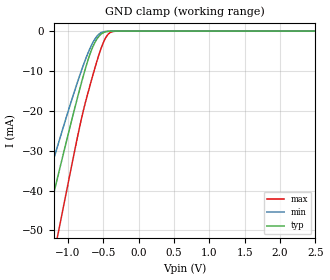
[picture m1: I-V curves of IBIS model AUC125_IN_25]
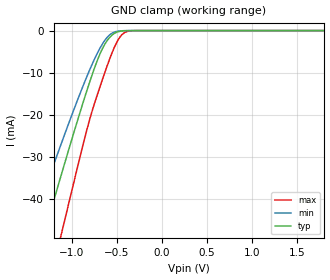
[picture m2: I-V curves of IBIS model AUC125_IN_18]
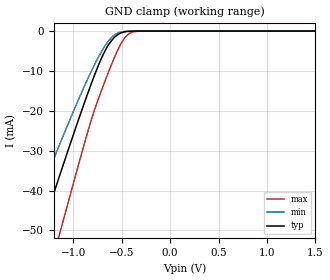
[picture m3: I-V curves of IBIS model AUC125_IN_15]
| TEXAS INSTRUMENTS INCORPORATED
| Standard Linear and Logic Group
| IBIS Model of SN74AUC125
| Quadruple Bus Buffer Gate with 3-state Outputs
| This file contains package information for the following:
|  QFN 14-pin (RGY) package as [Component] AUC125_RGY
| This device can be powered at the following Vccs:
|  2.5 volt Vcc
|  1.8 volt Vcc
|  1.5 volt Vcc
|  1.2 volt Vcc
|  0.8 volt Vcc
| This file provides unique models under the [Model Selector] for each Vcc.
| For operation at a specific Vcc, select the appropriate model after each
| [Model Selector] keyword.
[IBIS Ver]   3.2
[Comment char]  |_char
[File Name]   sn74auc125.ibs
[File Rev]   1.1 | x_die
[Date]   September 12, 2003
[Source]   Data created from TI-SPICE simulations at TI-SLL.
[Notes]   The following is an IBIS list for the AUC125.
   Please contact sllibis@ti.com with questions and
   comments concerning SLL IBIS models.
   - Power clamp data deleted as there is no power-clamp diode.
   - End point warning due to AC and DC mismatch.
   - Non-monotonic data in pullup and pulldown due to
   feedback circuit.
[Disclaimer] Property of Texas Instruments Incorporated.  Unauthorized
   reproduction and/or distribution is strictly prohibited.
   This product is protected under copyright law.
   Created  2003, (C) Copyright  2003, Texas Instruments
   Incorporated, All Rights Reserved
   UNLESS THERE IS A SIGNED, WRITTEN AGREEMENT TO THE
   CONTRARY, TEXAS INSTRUMENTS (TI) IS PROVIDING THE IBIS
   MODELS  AND WITHOUT ANY WARRANTY, EXPRESSED OR
   IMPLIED.  TI assumes no liability for:
   1) the accuracy of the IBIS models provided to your
   company;
   2) the proper functioning of these IBIS Models in your
   design or for any resulting applications; or
   3) infringement of patents, copyrights or intellectual
   property rights resulting from your use of these IBIS
   models.
   TI provides IBIS Models as a service to our customers.
   You and your company shall not distribute, sell or give
   these models to anyone else without prior written
   permission from TI.
   TI reserves the right to make changes to our products or
   to discontinue any semiconductor product or service
   without notice, and advises our customers to obtain the
   latest version of relevant information to verify, before
   placing orders, that the information being relied on is
   current.
   Please be aware that your receipt and use of the IBIS
   information provided shall serve as acceptance of these
   terms and conditions.  If you do not accept these terms,
   you should return or destroy the IBIS models and any
   other accompanying information immediately.
| Component AUC125_RGY 14-pin QFN
[Component]   AUC125_RGY
[Manufacturer]   Texas Instruments, Inc.
[Package]
|   typ   min   max
R_pkg   2.900e-02   2.300e-02   4.100e-02
L_pkg   7.730e-10   6.570e-10   9.980e-10
C_pkg   1.360e-13   1.150e-13   1.560e-13
[Pin]   signal_name   model_name   R_pin   L_pin   C_pin
1   1NOE   AUC125_IN_OE   2.700e-02   8.310e-10   1.300e-13
2   1A   AUC125_IN   2.700e-02   8.660e-10   1.350e-13
3   1Y   AUC125_OUT   4.100e-02   9.980e-10   1.560e-13
4   2NOE   AUC125_IN_OE   3.100e-02   7.670e-10   1.420e-13
5   2A   AUC125_IN   3.100e-02   7.650e-10   1.420e-13
6   2Y   AUC125_OUT   3.100e-02   7.830e-10   1.440e-13
7   GND   GND   3.100e-02   7.810e-10   1.370e-13
8   3Y   AUC125_OUT   2.300e-02   6.570e-10   1.150e-13
9   3A   AUC125_IN   2.300e-02   8.140e-10   1.290e-13
10   3NOE   AUC125_IN_OE   2.800e-02   7.040e-10   1.290e-13
11   4Y   AUC125_OUT   2.700e-02   6.720e-10   1.360e-13
12   4A   AUC125_IN   2.700e-02   6.960e-10   1.380e-13
13   4NOE   AUC125_IN_OE   2.700e-02   7.250e-10   1.400e-13
14   VCC   POWER   3.000e-02   7.630e-10   1.360e-13
| Model AUC125_IN
[Model Selector]   AUC125_IN
AUC125_IN_25   2.5 volt Vcc
AUC125_IN_18   1.8 volt Vcc
AUC125_IN_15   1.5 volt Vcc
AUC125_IN_12   1.2 volt Vcc
AUC125_IN_08   0.8 volt Vcc
| Model AUC125_IN_OE
[Model Selector]   AUC125_IN_OE
AUC125_IN_OE_25   2.5 volt Vcc
AUC125_IN_OE_18   1.8 volt Vcc
AUC125_IN_OE_15   1.5 volt Vcc
AUC125_IN_OE_12   1.2 volt Vcc
AUC125_IN_OE_08   0.8 volt Vcc
| Model AUC125_OUT
[Model Selector]   AUC125_OUT
AUC125_OUT_25   2.5 volt Vcc
AUC125_OUT_18   1.8 volt Vcc
AUC125_OUT_15   1.5 volt Vcc
AUC125_OUT_12   1.2 volt Vcc
AUC125_OUT_08   0.8 volt Vcc
| Models and submodels in the file (15): AUC125_IN_25 (Input), AUC125_IN_18 (Input), AUC125_IN_15 (Input), AUC125_IN_12 (Input), AUC125_IN_08 (Input), AUC125_IN_OE_25 (Input), AUC125_IN_OE_18 (Input), AUC125_IN_OE_15 (Input), AUC125_IN_OE_12 (Input), AUC125_IN_OE_08 (Input), AUC125_OUT_25 (3-state), AUC125_OUT_18 (3-state), AUC125_OUT_15 (3-state), AUC125_OUT_12 (3-state), AUC125_OUT_08 (3-state)
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[Model]   AUC125_IN_25
Model_type  Input
Vinl=0.7
Vinh=1.7
| variable   typ   min   max
C_comp   2.25pF   1.80pF   2.70pF
[Temperature Range]   40   100   -40
| Ambient temperature   25   85   -40
[Voltage range]   2.5   2.3   2.7
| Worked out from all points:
|   GND clamp passes 1 mA (typ) near -0.55 V on its own axis
[GND Clamp]
| AUC125_IN_25
|   Voltage   I(typ)   I(min)   I(max)
-3.6V     -222.3mA   -186mA     -267.4mA
-1.49V    -62.27mA   -49.76mA   -82.08mA
-1.35V    -51.78mA   -41.12mA   -69.61mA
-1.305V   -48.43mA   -38.37mA   -65.59mA
-1.17V    -38.45mA   -30.23mA   -53.54mA
-1.12V    -34.78mA   -27.27mA   -49.07mA
-735mV    -8.323mA   -6.326mA   -16.67mA
-635mV    -3.426mA   -2.469mA   -10.25mA
-525mV    -682.5uA   -360.1uA   -4.021mA
-430mV    -73.19uA   -34.72uA   -776.9uA
-325mV    -3.339uA   -2.005uA   -30.74uA
2.5V      313.9pA    400.8pA    470.4pA
[Model]   AUC125_IN_18
Model_type  Input
Vinl=0.5775
Vinh=1.2675
| variable   typ   min   max
C_comp   2.32pF   1.89pF   2.71pF
[Temperature Range]   40   100   -40
| Ambient temperature   25   85   -40
[Voltage range]   1.8   1.65   1.95
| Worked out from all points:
|   GND clamp passes 1 mA (typ) near -0.55 V on its own axis
[GND Clamp]
| AUC125_IN_18
|   Voltage   I(typ)   I(min)   I(max)
-3.6V     -222.3mA   -186mA     -267.4mA
-1.475V   -61.14mA   -48.83mA   -80.75mA
-1.43V    -57.76mA   -46.04mA   -76.74mA
-1.295V   -47.69mA   -37.76mA   -64.7mA
-1.1V     -33.32mA   -26.09mA   -47.29mA
-830mV    -14.31mA   -10.95mA   -23.64mA
-680mV    -5.361mA   -4.028mA   -13.09mA
-560mV    -1.272mA   -753.1uA   -5.827mA
-485mV    -290.6uA   -140.1uA   -2.305mA
-420mV    -55.81uA   -26.71uA   -608.5uA
-300mV    -1.501uA   -987.4nA   -11.88uA
1.8V      203.2pA    297.2pA    235.5pA
[Model]   AUC125_IN_15
Model_type  Input
Vinl=0.49
Vinh=1.04
| variable   typ   min   max
C_comp   2.35pF   1.94pF   2.69pF
[Temperature Range]   40   100   -40
| Ambient temperature   25   85   -40
[Voltage range]   1.5   1.4   1.6
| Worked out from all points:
|   GND clamp passes 1 mA (typ) near -0.55 V on its own axis
[GND Clamp]
| AUC125_IN_15
|   Voltage   I(typ)   I(min)   I(max)
-3.6V     -222.3mA   -186mA     -267.4mA
-1.505V   -63.39mA   -50.69mA   -83.42mA
-1.325V   -49.92mA   -39.59mA   -67.38mA
-1.17V    -38.45mA   -30.23mA   -53.54mA
-1.12V    -34.78mA   -27.27mA   -49.07mA
-840mV    -14.97mA   -11.47mA   -24.46mA
-695mV    -6.113mA   -4.618mA   -14.06mA
-570mV    -1.487mA   -910.9uA   -6.381mA
-495mV    -364.6uA   -178.7uA   -2.692mA
-430mV    -73.19uA   -34.72uA   -776.9uA
-280mV    -781.4nA   -556.2nA   -5.358uA
1.5V      165.9pA    258.5pA    172.1pA
